(* Logix 5000 AddOnInstructionDefinition export NXEE2_Apply_Preset; software revision 20.05 *)

TYPE AMCI_NXEE2_Input_Data :
STRUCT
   Word_0_Reserved_Bit_0 : BOOL;
   Word_0_Reserved_Bit_1 : BOOL;
   CH1_Motion_Detection : BOOL;
   CH1_Velocity_at_Zero : BOOL;
   CH1_Command_Error : BOOL;
   CH1_Config_Error : BOOL;
   CH1_SSI_Setup_Error : BOOL;
   CH1_Scalar_Errors : BOOL;
   CH1_Preset_Value_Error : BOOL;
   CH1_FSC_Error : BOOL;
   CH1_FSC_Exceeded : BOOL;
   Memory_Error : BOOL;
   CH1_Input_State : BOOL;
   CH1_Value_Captured : BOOL;
   Heartbeat : BOOL;
   Acknowledge_Bit : BOOL;
   Word_1_Reserved_Bit_0 : BOOL;
   Word_1_Reserved_Bit_1 : BOOL;
   CH2_Motion_Detection : BOOL;
   CH2_Velocity_at_Zero : BOOL;
   CH2_Command_Error : BOOL;
   CH2_Config_Error : BOOL;
   CH2_SSI_Setup_Error : BOOL;
   CH2_Scalar_Errors : BOOL;
   CH2_Preset_Value_Error : BOOL;
   CH2_FSC_Error : BOOL;
   CH2_FSC_Exceeded : BOOL;
   Word_1_Reserved_bit_11 : BOOL;
   CH2_Input_State : BOOL;
   CH2_Value_Captured : BOOL;
   Word_1_Reserved_bit_14 : BOOL;
   Word_1_Reserved_bit_15 : BOOL;
   CH1_Value_1 : DINT;
   CH1_Value_2 : DINT;
   CH2_Value_1 : DINT;
   CH2_Value_2 : DINT;
END_STRUCT
END_TYPE

TYPE AMCI_NXEE2_Output_Data :
STRUCT
   Command_Word : INT;
   Configuration_Word : INT;
   Number_of_SSI_Data_Bits : INT;
   Number_Of_Data_Value_Bits : SINT;
   MSB_Number : SINT;
   Scalar_Multiplier : INT;
   Scalar_Divisor : INT;
   Preset_Value : DINT;
   Full_Scale_Count : DINT;
END_STRUCT
END_TYPE

ADD_ON_INSTRUCTION NXEE2_Apply_Preset   (* revision 2.0, vendor AMCI, ExecuteEnableInFalse *)
// Revision note:
// 1/29/21 Revision 1.0.  Initial release
// 12/18/2025: Revision 2.0.  Modified the AOIs to use User Defined Input and Output Data
VAR_IN_OUT
   NXEE2_Input_Data : AMCI_NXEE2_Input_Data; {required}
        .0   // set when command error
        .15   // ACK bit
        .2   // set when reference voltage error
        .3   // set when reference frequency error
        .4   // command error
        .5   // config error
        .6   // setup error
        .7   // scalar errors
        .8   // preset value error
        .9   // full scale count error
   NXEE2_Output_Data : AMCI_NXEE2_Output_Data; {required}
END_VAR
VAR_INPUT
   Apply_Preset_Ch1_0_NO_1_YES : BOOL; {required}
   Apply_Preset_Ch2_0_NO_1_YES : BOOL; {required}
   Save_In_Flash_0_NO_1_YES : BOOL; {required}
END_VAR
VAR_OUTPUT
   EN : BOOL; {access Read Only, visible}
   DN : BOOL; {access Read Only, visible}
   ER : BOOL; {visible}
END_VAR
VAR
   command_data_block : INT[10];
        [0]   // Command Word
        [0].15   // Transmit bit
        [1]   // Setup Word
        [2]   // channel 1 Full Scale_Count
        [3]   // channel 1 Preset Value
        [4]   // channel 1 Transformation Ratio
        [5]   // channel 2 Full Scale Count
        [6]   // channel 2 Preset Value
        [7]   // channel 2 Transformation Ratio
        [8]   // Reference Voltage
        [9]   // Reference Frequency
   Allow_Programming : BOOL; {access None}
END_VAR

ROUTINE EnableInFalse   (* ladder *)
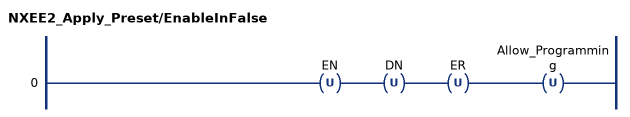
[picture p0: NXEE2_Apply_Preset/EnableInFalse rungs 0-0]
   0: OTU(EN)OTU(DN)OTU(ER)OTU(Allow_Programming);
END_ROUTINE

ROUTINE Logic   (* ladder *)
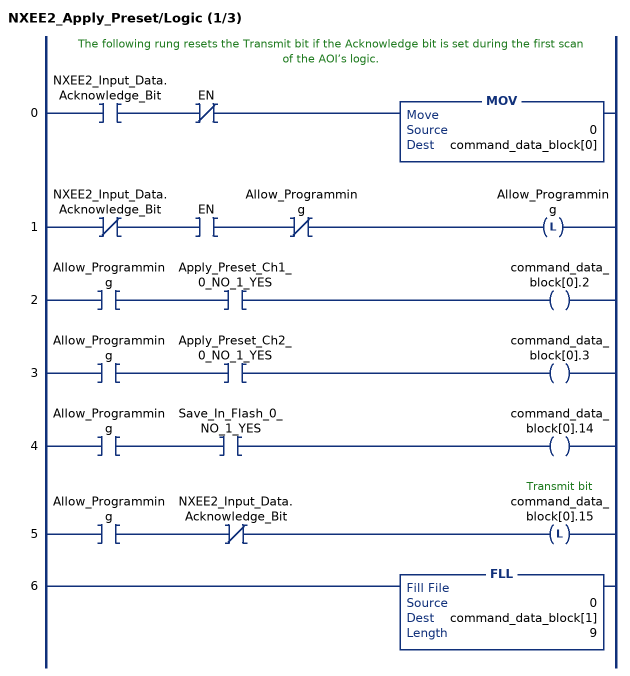
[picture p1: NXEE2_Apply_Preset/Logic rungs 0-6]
   // The following rung resets the Transmit bit if the Acknowledge bit is set during the first scan of the AOI’s logic.
   0: XIC(NXEE2_Input_Data.Acknowledge_Bit)XIO(EN)MOV(0,command_data_block[0]);
   1: XIO(NXEE2_Input_Data.Acknowledge_Bit)XIC(EN)XIO(Allow_Programming)OTL(Allow_Programming);
   2: XIC(Allow_Programming)XIC(Apply_Preset_Ch1_0_NO_1_YES)OTE(command_data_block[0].2);
   3: XIC(Allow_Programming)XIC(Apply_Preset_Ch2_0_NO_1_YES)OTE(command_data_block[0].3);
   4: XIC(Allow_Programming)XIC(Save_In_Flash_0_NO_1_YES)OTE(command_data_block[0].14);
   5: XIC(Allow_Programming)XIO(NXEE2_Input_Data.Acknowledge_Bit)OTL(command_data_block[0].15);
   6: FLL(0,command_data_block[1],9);
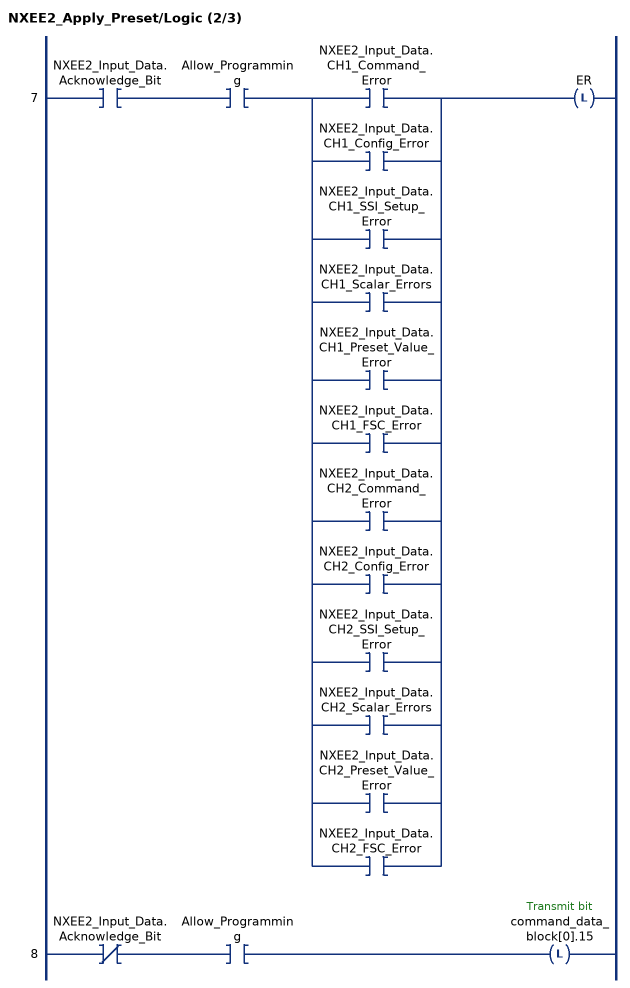
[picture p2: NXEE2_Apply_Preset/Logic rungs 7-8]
   7: XIC(NXEE2_Input_Data.Acknowledge_Bit)XIC(Allow_Programming)[XIC(NXEE2_Input_Data.CH1_Command_Error) ,XIC(NXEE2_Input_Data.CH1_Config_Error) ,XIC(NXEE2_Input_Data.CH1_SSI_Setup_Error) ,XIC(NXEE2_Input_Data.CH1_Scalar_Errors) ,XIC(NXEE2_Input_Data.CH1_Preset_Value_Error) ,XIC(NXEE2_Input_Data.CH1_FSC_Error) ,XIC(NXEE2_Input_Data.CH2_Command_Error) ,XIC(NXEE2_Input_Data.CH2_Config_Error) ,XIC(NXEE2_Input_Data.CH2_SSI_Setup_Error) ,XIC(NXEE2_Input_Data.CH2_Scalar_Errors) ,XIC(NXEE2_Input_Data.CH2_Preset_Value_Error) ,XIC(NXEE2_Input_Data.CH2_FSC_Error) ]OTL(ER);
   8: XIO(NXEE2_Input_Data.Acknowledge_Bit)XIC(Allow_Programming)OTL(command_data_block[0].15);
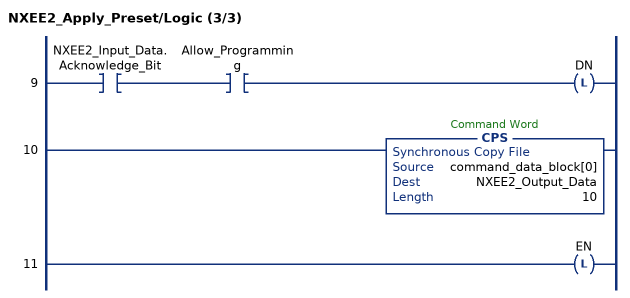
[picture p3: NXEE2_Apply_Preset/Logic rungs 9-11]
   9: XIC(NXEE2_Input_Data.Acknowledge_Bit)XIC(Allow_Programming)OTL(DN);
   10: CPS(command_data_block[0],NXEE2_Output_Data,10);
   11: OTL(EN);
END_ROUTINE
END_ADD_ON_INSTRUCTION
